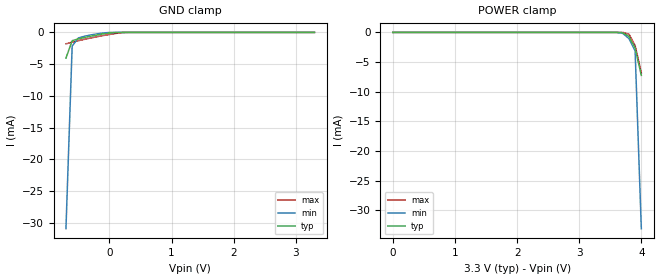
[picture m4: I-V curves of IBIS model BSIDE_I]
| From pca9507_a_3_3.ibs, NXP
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[Model]   BSIDE_I
Model_type Input
Vinh=2.31
Vinl=0.99
C_comp   4.8p   4.6p   5p
[Temperature Range] 27   85   -40
[Voltage Range]   3.3   3   3.6
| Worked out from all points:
|   GND clamp passes 1 mA (typ) near -0.49 V on its own axis
[GND Clamp]
-700mV    -4.05mA    -30.95mA   -1.806mA
-600mV    -1.31mA    -2.161mA   -1.533mA
-500mV    -1.019mA   -875.3uA   -1.302mA
-100mV    -246.1uA   -93.43uA   -501.2uA
100mV     -17.77uA   -705.6nA   -166.7uA
300mV     -12.16nA   -372.9pA   -1.544uA
3.3V      175.6pA    197.3pA    170.4pA
[POWER Clamp]
0V        211.3pA    369.9pA    198.3pA
3.5V      -25.4nA    -195.4nA   -672.8pA
3.7V      -54.36uA   -160.3uA   -7.617uA
3.8V      -661uA     -1.03mA    -281.8uA
3.9V      -2.648mA   -3.107mA   -2.21mA
4V        -7.254mA   -33.12mA   -6.833mA
